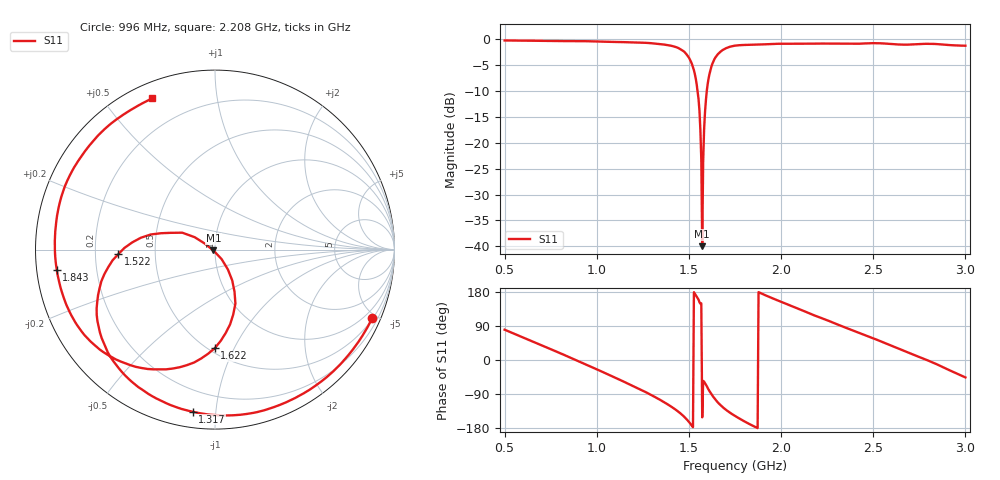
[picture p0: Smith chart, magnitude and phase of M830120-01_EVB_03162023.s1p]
# Hz S RI R 50
! CMT, M5090, 19127454, 21.2.4/2
! Date: 3/16/2023 5:30:30 PM
! Data: Format (Calibration Info)
! Freq	S11:Re/Im(F2)
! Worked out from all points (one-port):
!   500 points, 500 MHz to 3 GHz, reference 50 ohm
!   lowest |S11| = -40.0 dB at 1.572 GHz (marker M1), VSWR 1.02, Z = 49.1 - j0.473 ohm
!   |S11| at or under -10 dB: 1.547 GHz to 1.597 GHz (49.94 MHz wide, 3.18 % of centre)
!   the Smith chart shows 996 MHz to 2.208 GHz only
!   S11 on the Smith chart (normalised r, x): 996 MHz: 0.54, -4.73; 1.317 GHz: 0.08, -0.87; 1.522 GHz: 0.30, -0.02; 1.622 GHz: 0.54, -0.84; 1.843 GHz: 0.06, -0.06; 2.208 GHz: 0.07, +0.67
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5e8  0.1705 0.9624
6.402806e8  0.6077 0.7582
8.156313e8  0.9308 0.2485
9.95992e8  0.8757 -0.3821
1.126253e9  0.5737 -0.7484
1.226453e9  0.235 -0.9053
1.316633e9  -0.1247 -0.9031
1.441884e9  -0.5976 -0.5719
1.486974e9  -0.656 -0.2909
1.522044e9  -0.5388 -0.0253
1.547094e9  -0.3007 0.0913
1.557114e9  -0.1824 0.0942
1.562124e9  -0.1137 0.0693
1.572144e9  -0.0088 -0.00481
1.582164e9  0.0719 -0.1109
1.587174e9  0.0961 -0.1721
1.597194e9  0.1138 -0.3004
1.622244e9  -0.000868 -0.5489
1.672345e9  -0.3758 -0.6651
1.752505e9  -0.7419 -0.4576
1.842685e9  -0.8814 -0.1142
2.063126e9  -0.7084 0.569
2.208417e9  -0.3498 0.8421
2.378758e9  0.1599 0.8936
2.519038e9  0.5461 0.74
2.689379e9  0.8404 0.295
2.834669e9  0.8927 -0.1429
3e9  0.604 -0.6252
